FUNCTION "MAGNETI AUSILIARI" : VOID
TITLE =
//BRUNO ANGELO E4.6 INGR. CON VENE 19 PONTICELLATE memorizzazione tav 1-2
AUTHOR : BRUNO
NAME : LAGON
VERSION : 0.1

BEGIN
NETWORK
TITLE =memorizzazione tav 1
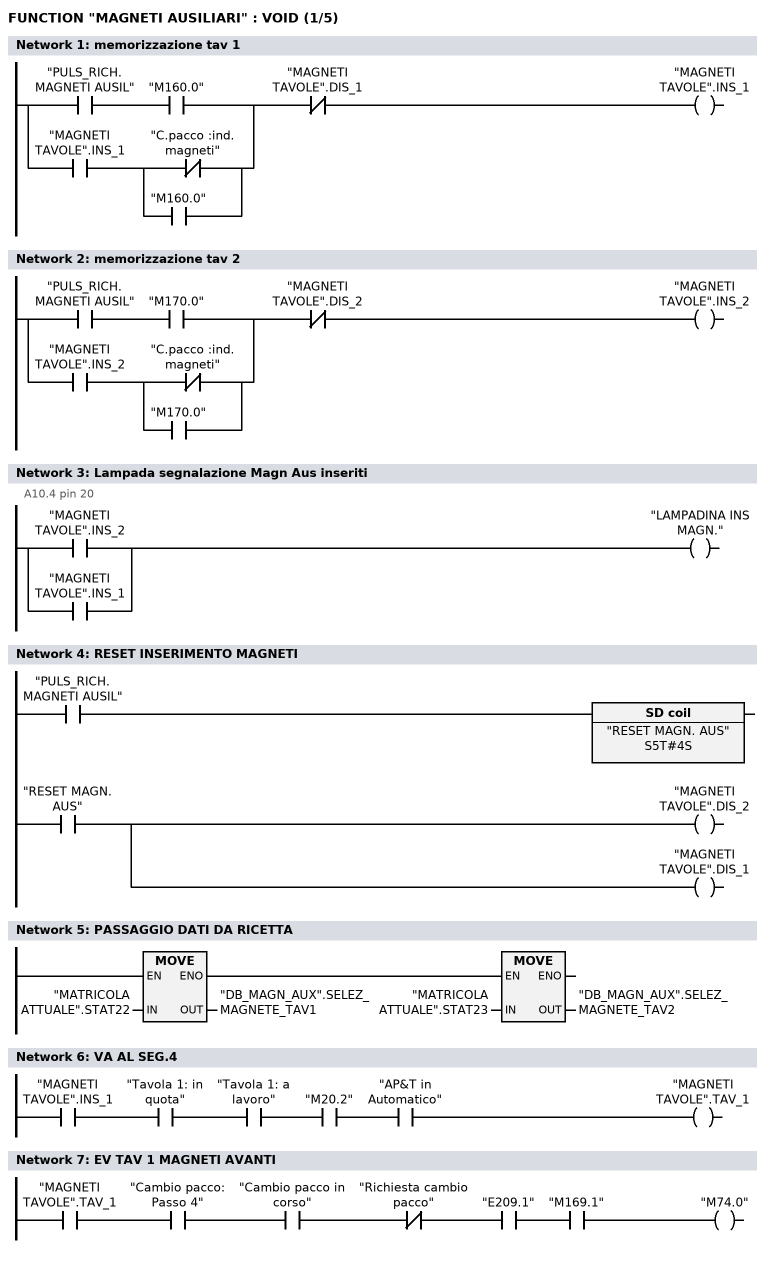
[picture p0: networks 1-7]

      U(    ;
      U     "PULS_RICH. MAGNETI AUSIL";
      U     "M160.0";
      O     ;
      U     "MAGNETI TAVOLE".INS_1;
      U(    ;
      ON    "C.pacco :ind. magneti";
      O     "M160.0";
      )     ;
      )     ;
      UN    "MAGNETI TAVOLE".DIS_1;
      =     "MAGNETI TAVOLE".INS_1;
NETWORK
TITLE =memorizzazione tav 2

      U(    ;
      U     "PULS_RICH. MAGNETI AUSIL";
      U     "M170.0";
      O     ;
      U     "MAGNETI TAVOLE".INS_2;
      U(    ;
      ON    "C.pacco :ind. magneti";
      O     "M170.0";
      )     ;
      )     ;
      UN    "MAGNETI TAVOLE".DIS_2;
      =     "MAGNETI TAVOLE".INS_2;
NETWORK
TITLE =Lampada segnalazione Magn Aus inseriti
//A10.4 pin 20
      O     "MAGNETI TAVOLE".INS_2;
      O     "MAGNETI TAVOLE".INS_1;
      =     "LAMPADINA INS MAGN.";
NETWORK
TITLE =RESET INSERIMENTO MAGNETI

      U     "PULS_RICH. MAGNETI AUSIL";
      L     S5T#4S;
      SE    "RESET MAGN. AUS";
      NOP   0;
      NOP   0;
      NOP   0;
      U     "RESET MAGN. AUS";
      =     "MAGNETI TAVOLE".DIS_2;
      =     "MAGNETI TAVOLE".DIS_1;
NETWORK
TITLE =PASSAGGIO DATI DA RICETTA

      U(    ;
      L     "MATRICOLA ATTUALE".STAT22;
      T     "DB_MAGN_AUX".SELEZ_MAGNETE_TAV1;
      SET   ;
      SAVE  ;
      CLR   ;
      U     BIE;
      )     ;
      SPBNB _001;
      L     "MATRICOLA ATTUALE".STAT23;
      T     "DB_MAGN_AUX".SELEZ_MAGNETE_TAV2;
_001: NOP   0;
NETWORK
TITLE =VA AL SEG.4

      U     "MAGNETI TAVOLE".INS_1;
      U     "Tavola 1: in quota";
      U     "Tavola 1: a  lavoro";
      U     "M20.2";
      U     "AP&T in Automatico";
      =     "MAGNETI TAVOLE".TAV_1;
NETWORK
TITLE =EV TAV 1 MAGNETI AVANTI

      U     "MAGNETI TAVOLE".TAV_1;
      U     "Cambio pacco: Passo 4";
      U     "Cambio pacco in corso";
      UN    "Richiesta cambio pacco";
      U     "E209.1";
      U     "M169.1";
      =     "M74.0";
NETWORK
TITLE ="TAV 1 MAGN IND"
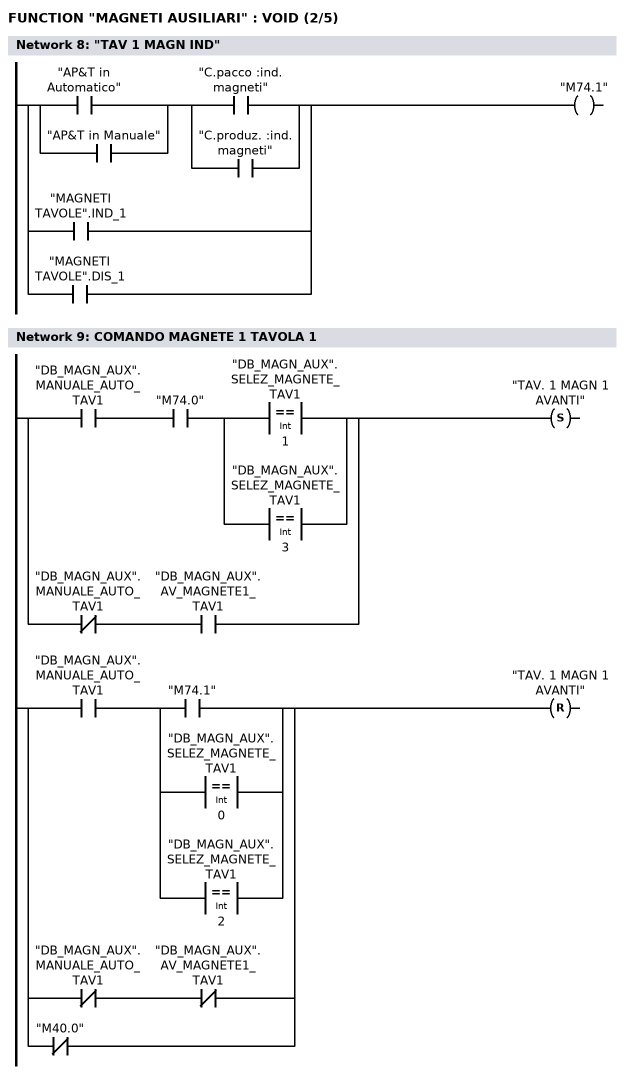
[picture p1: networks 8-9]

      U(    ;
      O     "AP&T in Automatico";
      O     "AP&T in Manuale";
      )     ;
      U(    ;
      O     "C.pacco :ind. magneti";
      O     "C.produz. :ind. magneti";
      )     ;
      O     "MAGNETI TAVOLE".IND_1;
      O     "MAGNETI TAVOLE".DIS_1;
      =     "M74.1";
NETWORK
TITLE =COMANDO MAGNETE 1 TAVOLA 1

      U(    ;
      U     "DB_MAGN_AUX".MANUALE_AUTO_TAV1;
      U     "M74.0";
      U(    ;
      O(    ;
      L     "DB_MAGN_AUX".SELEZ_MAGNETE_TAV1;
      L     1;
      ==I   ;
      )     ;
      O(    ;
      L     "DB_MAGN_AUX".SELEZ_MAGNETE_TAV1;
      L     3;
      ==I   ;
      )     ;
      )     ;
      O     ;
      UN    "DB_MAGN_AUX".MANUALE_AUTO_TAV1;
      U     "DB_MAGN_AUX".AV_MAGNETE1_TAV1;
      )     ;
      S     "TAV. 1 MAGN  1  AVANTI";
      U(    ;
      U     "DB_MAGN_AUX".MANUALE_AUTO_TAV1;
      U(    ;
      O     "M74.1";
      O(    ;
      L     "DB_MAGN_AUX".SELEZ_MAGNETE_TAV1;
      L     0;
      ==I   ;
      )     ;
      O(    ;
      L     "DB_MAGN_AUX".SELEZ_MAGNETE_TAV1;
      L     2;
      ==I   ;
      )     ;
      )     ;
      O     ;
      UN    "DB_MAGN_AUX".MANUALE_AUTO_TAV1;
      UN    "DB_MAGN_AUX".AV_MAGNETE1_TAV1;
      ON    "M40.0";
      )     ;
      R     "TAV. 1 MAGN  1  AVANTI";
      NOP   0;
NETWORK
TITLE =COMANDO MAGNETE 2 TAVOLA 1
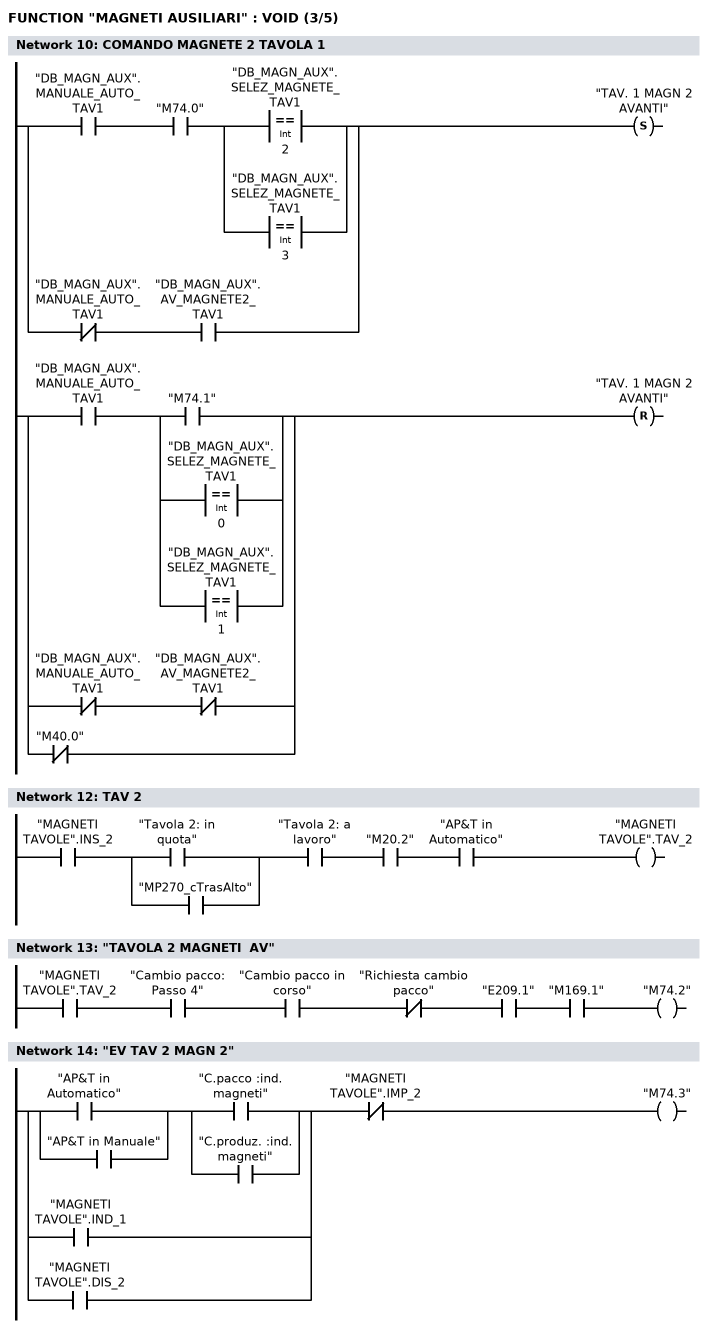
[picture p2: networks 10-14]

      U(    ;
      U     "DB_MAGN_AUX".MANUALE_AUTO_TAV1;
      U     "M74.0";
      U(    ;
      O(    ;
      L     "DB_MAGN_AUX".SELEZ_MAGNETE_TAV1;
      L     2;
      ==I   ;
      )     ;
      O(    ;
      L     "DB_MAGN_AUX".SELEZ_MAGNETE_TAV1;
      L     3;
      ==I   ;
      )     ;
      )     ;
      O     ;
      UN    "DB_MAGN_AUX".MANUALE_AUTO_TAV1;
      U     "DB_MAGN_AUX".AV_MAGNETE2_TAV1;
      )     ;
      S     "TAV. 1 MAGN  2  AVANTI";
      U(    ;
      U     "DB_MAGN_AUX".MANUALE_AUTO_TAV1;
      U(    ;
      O     "M74.1";
      O(    ;
      L     "DB_MAGN_AUX".SELEZ_MAGNETE_TAV1;
      L     0;
      ==I   ;
      )     ;
      O(    ;
      L     "DB_MAGN_AUX".SELEZ_MAGNETE_TAV1;
      L     1;
      ==I   ;
      )     ;
      )     ;
      O     ;
      UN    "DB_MAGN_AUX".MANUALE_AUTO_TAV1;
      UN    "DB_MAGN_AUX".AV_MAGNETE2_TAV1;
      ON    "M40.0";
      )     ;
      R     "TAV. 1 MAGN  2  AVANTI";
      NOP   0;
NETWORK
TITLE =

NETWORK
TITLE =TAV 2

      U     "MAGNETI TAVOLE".INS_2;
      U(    ;
      O     "Tavola 2: in quota";
      O     "MP270_cTrasAlto";
      )     ;
      U     "Tavola 2: a  lavoro";
      U     "M20.2";
      U     "AP&T in Automatico";
      =     "MAGNETI TAVOLE".TAV_2;
NETWORK
TITLE ="TAVOLA 2 MAGNETI  AV"

      U     "MAGNETI TAVOLE".TAV_2;
      U     "Cambio pacco: Passo 4";
      U     "Cambio pacco in corso";
      UN    "Richiesta cambio pacco";
      U     "E209.1";
      U     "M169.1";
      =     "M74.2";
NETWORK
TITLE ="EV TAV 2 MAGN 2"

      U(    ;
      U(    ;
      O     "AP&T in Automatico";
      O     "AP&T in Manuale";
      )     ;
      U(    ;
      O     "C.pacco :ind. magneti";
      O     "C.produz. :ind. magneti";
      )     ;
      O     "MAGNETI TAVOLE".IND_1;
      O     "MAGNETI TAVOLE".DIS_2;
      )     ;
      UN    "MAGNETI TAVOLE".IMP_2;
      =     "M74.3";
NETWORK
TITLE =COMANDO MAGNETE 1 TAVOLA 2
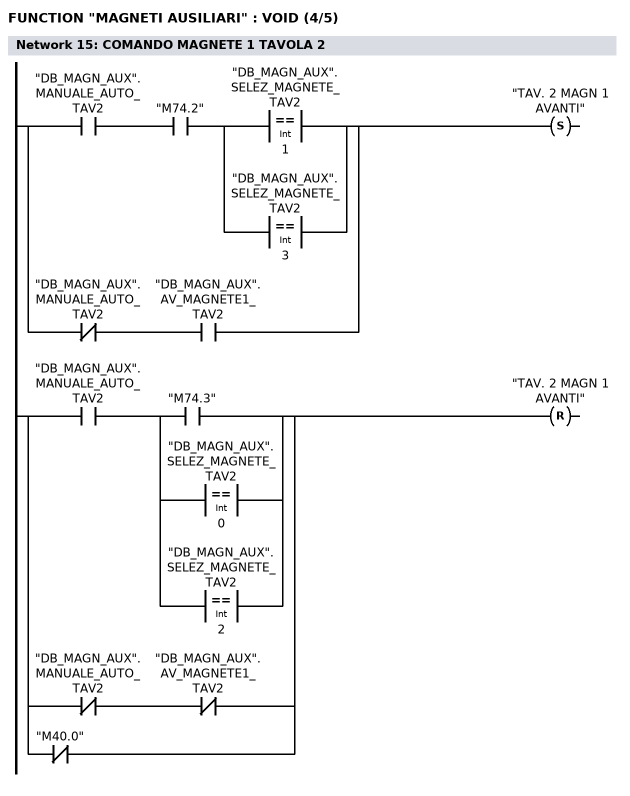
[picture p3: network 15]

      U(    ;
      U     "DB_MAGN_AUX".MANUALE_AUTO_TAV2;
      U     "M74.2";
      U(    ;
      O(    ;
      L     "DB_MAGN_AUX".SELEZ_MAGNETE_TAV2;
      L     1;
      ==I   ;
      )     ;
      O(    ;
      L     "DB_MAGN_AUX".SELEZ_MAGNETE_TAV2;
      L     3;
      ==I   ;
      )     ;
      )     ;
      O     ;
      UN    "DB_MAGN_AUX".MANUALE_AUTO_TAV2;
      U     "DB_MAGN_AUX".AV_MAGNETE1_TAV2;
      )     ;
      S     "TAV. 2 MAGN  1  AVANTI";
      U(    ;
      U     "DB_MAGN_AUX".MANUALE_AUTO_TAV2;
      U(    ;
      O     "M74.3";
      O(    ;
      L     "DB_MAGN_AUX".SELEZ_MAGNETE_TAV2;
      L     0;
      ==I   ;
      )     ;
      O(    ;
      L     "DB_MAGN_AUX".SELEZ_MAGNETE_TAV2;
      L     2;
      ==I   ;
      )     ;
      )     ;
      O     ;
      UN    "DB_MAGN_AUX".MANUALE_AUTO_TAV2;
      UN    "DB_MAGN_AUX".AV_MAGNETE1_TAV2;
      ON    "M40.0";
      )     ;
      R     "TAV. 2 MAGN  1  AVANTI";
      NOP   0;
NETWORK
TITLE =COMANDO MAGNETE 2 TAVOLA 1
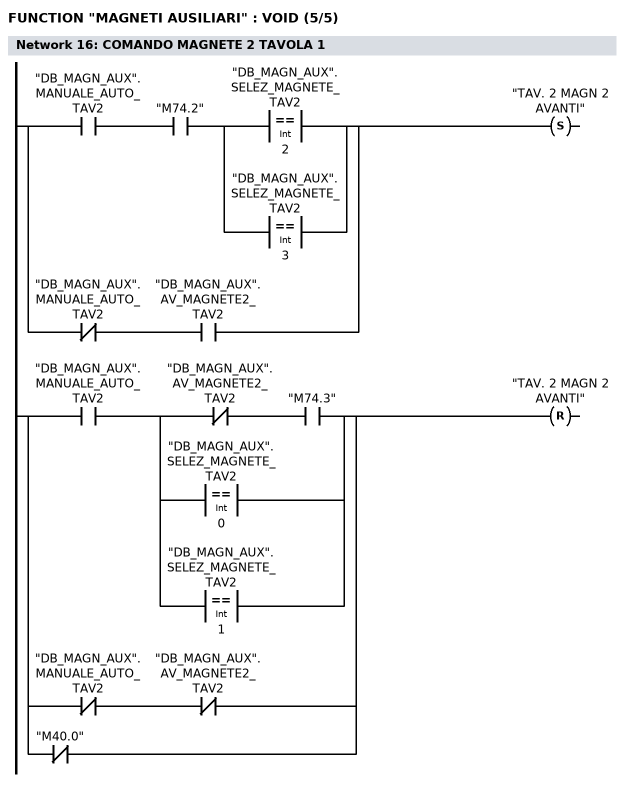
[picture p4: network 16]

      U(    ;
      U     "DB_MAGN_AUX".MANUALE_AUTO_TAV2;
      U     "M74.2";
      U(    ;
      O(    ;
      L     "DB_MAGN_AUX".SELEZ_MAGNETE_TAV2;
      L     2;
      ==I   ;
      )     ;
      O(    ;
      L     "DB_MAGN_AUX".SELEZ_MAGNETE_TAV2;
      L     3;
      ==I   ;
      )     ;
      )     ;
      O     ;
      UN    "DB_MAGN_AUX".MANUALE_AUTO_TAV2;
      U     "DB_MAGN_AUX".AV_MAGNETE2_TAV2;
      )     ;
      S     "TAV. 2 MAGN  2  AVANTI";
      U(    ;
      U     "DB_MAGN_AUX".MANUALE_AUTO_TAV2;
      U(    ;
      UN    "DB_MAGN_AUX".AV_MAGNETE2_TAV2;
      U     "M74.3";
      O(    ;
      L     "DB_MAGN_AUX".SELEZ_MAGNETE_TAV2;
      L     0;
      ==I   ;
      )     ;
      O(    ;
      L     "DB_MAGN_AUX".SELEZ_MAGNETE_TAV2;
      L     1;
      ==I   ;
      )     ;
      )     ;
      O     ;
      UN    "DB_MAGN_AUX".MANUALE_AUTO_TAV2;
      UN    "DB_MAGN_AUX".AV_MAGNETE2_TAV2;
      ON    "M40.0";
      )     ;
      R     "TAV. 2 MAGN  2  AVANTI";
      NOP   0;
END_FUNCTION

